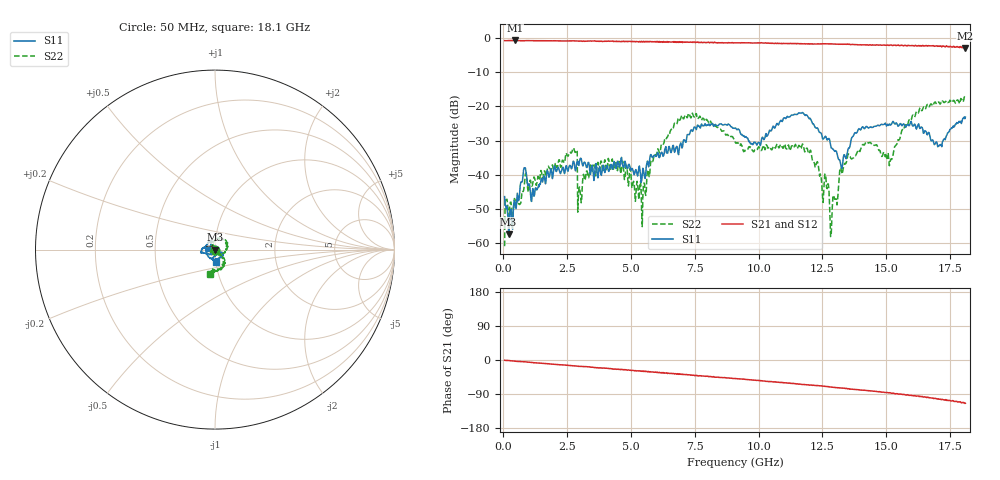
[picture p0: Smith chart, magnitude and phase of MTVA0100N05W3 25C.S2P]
! Network Analyzer HP8720D.06.14 Serial No. US36140669
! 17 Jan 2005  08:50:33
! Frequency  S11  S21  S12  S22
# HZ  S  DB R 50
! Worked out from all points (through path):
!   801 points, 50 MHz to 18.1 GHz, reference 50 ohm
!   highest |S21| = -0.71 dB at 456.1 MHz (marker M1); lowest = -2.9 dB at 18.1 GHz (marker M2)
!   group delay of S21, straight-line fit = 16.5 ps
!   lowest |S11| = -57.4 dB at 207.9 MHz (marker M3), VSWR 1.00, Z = 50.1 - j0.000728 ohm
!   |S11| at or under -10 dB: start of sweep to end of sweep
!   |S22| runs from -60.8 to -17.1 dB; largest |S21 - S12| = 0.029
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5e7  -46.32 -65.6  -0.76 -0.7  -0.75 -1.1  -60.79 -72.2
2.079375e8  -57.38 -0.3  -0.74 -1.3  -0.73 -1.5  -51.70 -8.2
4.56125e8  -47.87 38.3  -0.71 -3.0  -0.73 -3.2  -47.14 0.1
8.17125e8  -37.87 39.8  -0.79 -4.9  -0.77 -5.1  -43.09 -57.7
1.155562e9  -43.98 37.2  -0.77 -6.7  -0.76 -7.1  -42.29 131.1
2.689812e9  -37.93 61.7  -0.82 -15.0  -0.84 -15.3  -33.24 116.6
3.073375e9  -36.18 76.3  -0.89 -17.0  -0.87 -17.3  -46.48 -138.7
4.336875e9  -36.06 47.1  -0.96 -23.6  -0.93 -24.0  -38.50 137.7
5.510125e9  -39.59 160.4  -1.08 -30.6  -1.11 -30.6  -42.31 152.4
6.074188e9  -33.71 -144.7  -1.16 -33.7  -1.16 -33.7  -32.67 125.9
7.202312e9  -28.22 127.8  -1.14 -38.9  -1.19 -39.4  -23.30 44.2
9.075e9  -26.34 -179.5  -1.40 -48.8  -1.39 -49.2  -30.20 -60.1
1.000006e10  -30.49 -179.1  -1.46 -54.3  -1.44 -54.5  -31.77 -64.5
1.209838e10  -24.72 -159.4  -1.69 -66.7  -1.73 -66.9  -35.44 167.4
1.266244e10  -29.45 -132.5  -1.69 -70.1  -1.72 -70.4  -43.70 139.9
1.28655e10  -32.15 -121.2  -1.75 -71.6  -1.71 -72.1  -53.34 85.4
1.351981e10  -32.17 -151.5  -1.84 -75.7  -1.83 -76.1  -33.83 -43.4
1.428694e10  -26.21 -169.8  -2.06 -81.2  -2.03 -81.1  -30.60 -100.2
1.509919e10  -25.49 -110.3  -2.16 -86.8  -2.08 -87.3  -35.60 -94.5
1.597912e10  -24.36 -47.8  -2.21 -93.1  -2.26 -94.2  -23.89 -45.0
1.708469e10  -31.27 -61.1  -2.40 -103.5  -2.26 -104.1  -19.06 -81.7
1.81e10  -23.11 -83.7  -2.92 -114.2  -2.80 -114.9  -17.15 -101.3
